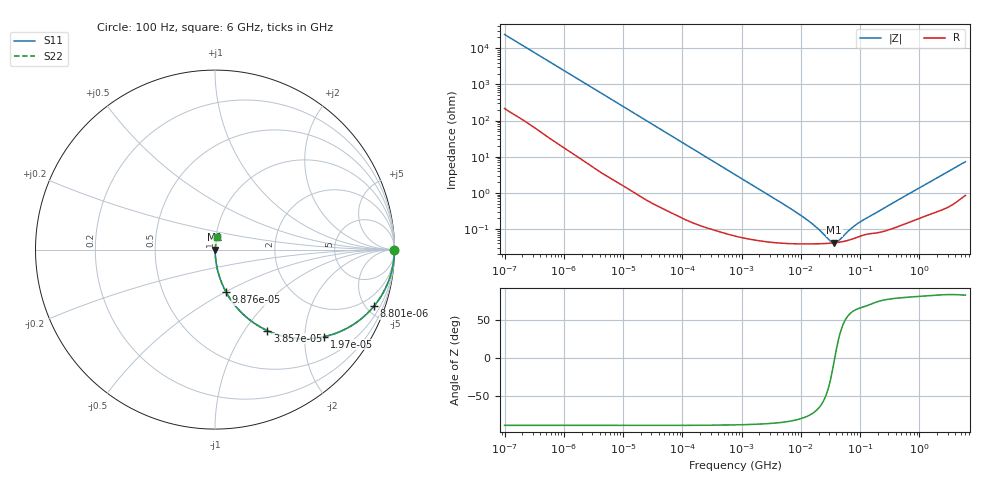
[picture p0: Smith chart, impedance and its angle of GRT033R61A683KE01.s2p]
!Murata Part Number: GRT033R61A683KE01
!These Parameters are Measured in Series Mode Connection
!Data Generated on Jun 19, 2026
!  o--ll--o
!Port1  Port2
!  o------o
!Operation Temp=25[degC], DC Bias Voltage=0[V]
!Freq. Start=100[Hz] Stop=6[GHz] 401[Steps]
# Hz S RI R 50
!Freq.(Hz) S11(Real) S11(Imag) S21(Real) S21(Imag) S12(Real) S12(Imag) S22(Real) S22(Imag)
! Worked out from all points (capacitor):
!   401 points, 100 Hz to 6 GHz, reference 50 ohm
!   read as one part in series: C = 66 nF near 109 Hz
!   lowest |Z| = 41.6 mohm at 36.42 MHz (marker M1)
!   series resonance near 37.42 MHz, so ESL is about 270 pH
!   S11 on the Smith chart (normalised r, x): 100 Hz: open; 8.801 kHz: 1.04, -5.59; 19.7 kHz: 1.02, -2.50; 38.57 kHz: 1.01, -1.28; 98.76 kHz: 1.00, -0.50; 6 GHz: 1.02, +0.14
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100  0.9999 -0.00415  5.44e-05 0.00415  5.44e-05 0.00415  0.9999 -0.00415
627  0.9991 -0.0258  0.000859 0.0258  0.000859 0.0258  0.9991 -0.0258
2008  0.9927 -0.0815  0.00725 0.0815  0.00725 0.0815  0.9927 -0.0815
4918  0.9602 -0.1923  0.0398 0.1923  0.0398 0.1923  0.9602 -0.1923
8801  0.8848 -0.3161  0.1152 0.3161  0.1152 0.3161  0.8848 -0.3161
13169  0.7761 -0.4137  0.2239 0.4137  0.2239 0.4137  0.7761 -0.4137
19704  0.6096 -0.4847  0.3904 0.4847  0.3904 0.4847  0.6096 -0.4847
26957  0.4563 -0.4949  0.5437 0.4949  0.5437 0.4949  0.4563 -0.4949
38569  0.2924 -0.4515  0.7076 0.4515  0.7076 0.4515  0.2924 -0.4515
40335  0.2744 -0.4428  0.7256 0.4428  0.7256 0.4428  0.2744 -0.4428
60352  0.1459 -0.3493  0.8541 0.3493  0.8541 0.3493  0.1459 -0.3493
98762  0.061 -0.2354  0.939 0.2354  0.939 0.2354  0.061 -0.2354
241822  0.0116 -0.1016  0.9884 0.1016  0.9884 0.1016  0.0116 -0.1016
774597  0.00168 -0.0323  0.9983 0.0323  0.9983 0.0323  0.00168 -0.0323
6353432  0.00041 -0.00387  0.9996 0.00387  0.9996 0.00387  0.00041 -0.00387
1.555665e7  0.000389 -0.00134  0.9996 0.00134  0.9996 0.00134  0.000389 -0.00134
3.045065e7  0.000403 -0.000279  0.9996 0.000279  0.9996 0.000279  0.000403 -0.000279
3.64232e7  0.000414 -3.58e-05  0.9996 3.58e-05  0.9996 3.58e-05  0.000414 -3.58e-05
4.35672e7  0.000429 0.000205  0.9996 -0.000205  0.9996 -0.000205  0.000429 0.000205
9.326766e7  0.000607 0.00132  0.9994 -0.00132  0.9994 -0.00132  0.000607 0.00132
3.124326e8  0.000978 0.00452  0.999 -0.00452  0.999 -0.00452  0.000978 0.00452
6e9  0.0134 0.0703  0.9866 -0.0703  0.9866 -0.0703  0.0134 0.0703
